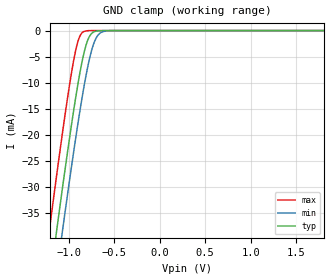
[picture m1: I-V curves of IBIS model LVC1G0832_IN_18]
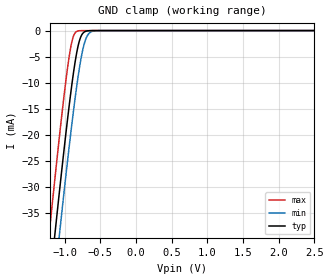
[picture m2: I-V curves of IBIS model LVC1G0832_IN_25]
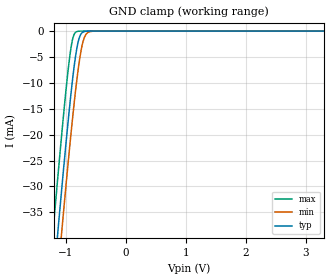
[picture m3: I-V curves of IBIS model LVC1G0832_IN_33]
| TEXAS INSTRUMENTS INCORPORATED
| Standard Linear and Logic Group
| IBIS Model of SN74LVC1G0832
| SINGLE 3-INPUT POSITIVE AND-OR GATE
| This file contains package information for the following:
|  SOT 5-pin (DBV) package as [Component] LVC1G0832_DBV
|  SOT 5-pin (DCK) package as [Component] LVC1G0832_DCK
|  NanoStar WCSP 5-pin (YEP) package as [Component] LVC1G0832_YEP
|  NanoFree WCSP 5-pin (YZP) package as [Component] LVC1G0832_YZP
| This device can be powered at the following Vccs:
|  1.8 volt Vcc
|  2.5 volt Vcc
|  3.3 volt Vcc
|  5 volt Vcc
| This file provides unique models under the [Model Selector] for each Vcc.
| For operation at a specific Vcc, select the appropriate model after each
| [Model Selector] keyword.
[IBIS Ver]   3.2
[Comment char]  |_char
[File Name]   sn74lvc1g0832.ibs
[File Rev]   1.2 | x_die
[Date]   August 4, 2005
[Source]   Data created from TI-SPICE simulations at TI-SLL.
[Notes]   The following is an IBIS list for the LVC1G0832.
   Please contact sllibis@ti.com with questions and
   comments concerning SLL IBIS models.
   - FILE REV HISTORY
   - 1.1 Release IBIS file on 10/04/04
   - 1.2 YEP and YZP packages added on 08/04/05
   - Due to the fact that the Device is 5.5-V Input tolarent,
   the pulldown model has some Non-Monotonic Warnings.
[Disclaimer] Property of Texas Instruments Incorporated.  Unauthorized
   reproduction and/or distribution is strictly prohibited.
   This product is protected under copyright law.
   Created  2004, (C) Copyright  2004, Texas Instruments
   Incorporated, All Rights Reserved
   UNLESS THERE IS A SIGNED, WRITTEN AGREEMENT TO THE
   CONTRARY, TEXAS INSTRUMENTS (TI) IS PROVIDING THE IBIS
   MODELS  AND WITHOUT ANY WARRANTY, EXPRESSED OR
   IMPLIED.  TI assumes no liability for:
   1) the accuracy of the IBIS models provided to your
   company;
   2) the proper functioning of these IBIS Models in your
   design or for any resulting applications; or
   3) infringement of patents, copyrights or intellectual
   property rights resulting from your use of these IBIS
   models.
   TI provides IBIS Models as a service to our customers.
   You and your company shall not distribute, sell or give
   these models to anyone else without prior written
   permission from TI.
   TI reserves the right to make changes to our products or
   to discontinue any semiconductor product or service
   without notice, and advises our customers to obtain the
   latest version of relevant information to verify, before
   placing orders, that the information being relied on is
   current.
   Please be aware that your receipt and use of the IBIS
   information provided shall serve as acceptance of these
   terms and conditions.  If you do not accept these terms,
   you should return or destroy the IBIS models and any
   other accompanying information immediately.
| Component LVC1G0832_DBV 5-pin SOT
[Component]   LVC1G0832_DBV
[Manufacturer]   Texas Instruments, Inc.
[Package]
|   typ   min   max
R_pkg   2.500e-02   1.900e-02   3.700e-02
L_pkg   1.524e-09   1.260e-09   1.751e-09
C_pkg   2.450e-13   1.980e-13   2.640e-13
[Pin]   signal_name   model_name   R_pin   L_pin   C_pin
1   A   LVC1G0832_IN   2.100e-02   1.405e-09   2.460e-13
2   B   LVC1G0832_IN   2.600e-02   1.493e-09   2.470e-13
3   GND   GND   3.700e-02   1.751e-09   2.630e-13
4   Y   LVC1G0832_OUT   1.900e-02   1.620e-09   2.640e-13
5   VCC   POWER   2.400e-02   1.260e-09   1.980e-13
| Component LVC1G0832_DCK 5-pin SOT
[Component]   LVC1G0832_DCK
[Manufacturer]   Texas Instruments, Inc.
[Package]
|   typ   min   max
R_pkg   2.500e-02   1.900e-02   3.700e-02
L_pkg   1.524e-09   1.260e-09   1.751e-09
C_pkg   2.450e-13   1.980e-13   2.640e-13
[Pin]   signal_name   model_name   R_pin   L_pin   C_pin
1   A   LVC1G0832_IN   2.100e-02   1.405e-09   2.460e-13
2   B   LVC1G0832_IN   2.600e-02   1.493e-09   2.470e-13
3   GND   GND   3.700e-02   1.751e-09   2.630e-13
4   Y   LVC1G0832_OUT   1.900e-02   1.620e-09   2.640e-13
5   VCC   POWER   2.400e-02   1.260e-09   1.980e-13
| Component LVC1G0832_YEP 5-pin NanoStar WCSP
[Component]   LVC1G0832_YEP
[Manufacturer]   Texas Instruments, Inc.
[Package]
|   typ   min   max
R_pkg   0.001   0.001   0.001
L_pkg   0.021nH   0.021nH   0.021nH
C_pkg   0.046pF   0.045pF   0.047pF
[Pin]   signal_name   model_name   R_pin   L_pin   C_pin
1   A   LVC1G0832_IN   0.001   0.021nH   0.046pF
2   B   LVC1G0832_IN   0.001   0.021nH   0.047pF
3   GND   GND   0.001   0.021nH   0.046pF
4   Y   LVC1G0832_OUT   0.001   0.021nH   0.045pF
5   VCC   POWER   0.001   0.021nH   0.045pF
| Component LVC1G0832_YZP 5-pin NanoStar WCSP
[Component]   LVC1G0832_YZP
[Manufacturer]   Texas Instruments, Inc.
[Package]
|   typ   min   max
R_pkg   0.001   0.001   0.001
L_pkg   0.021nH   0.021nH   0.021nH
C_pkg   0.046pF   0.045pF   0.047pF
[Pin]   signal_name   model_name   R_pin   L_pin   C_pin
1   A   LVC1G0832_IN   0.001   0.021nH   0.046pF
2   B   LVC1G0832_IN   0.001   0.021nH   0.047pF
3   GND   GND   0.001   0.021nH   0.046pF
4   Y   LVC1G0832_OUT   0.001   0.021nH   0.045pF
5   VCC   POWER   0.001   0.021nH   0.045pF
| Model LVC1G0832_IN
[Model Selector]   LVC1G0832_IN
LVC1G0832_IN_18   1.8 volt Vcc
LVC1G0832_IN_25   2.5 volt Vcc
LVC1G0832_IN_33   3.3 volt Vcc
LVC1G0832_IN_50   5 volt Vcc
| Model LVC1G0832_OUT
[Model Selector]   LVC1G0832_OUT
LVC1G0832_OUT_18   1.8 volt Vcc
LVC1G0832_OUT_25   2.5 volt Vcc
LVC1G0832_OUT_33   3.3 volt Vcc
LVC1G0832_OUT_50   5 volt Vcc
| Models and submodels in the file (8): LVC1G0832_IN_18 (Input), LVC1G0832_IN_25 (Input), LVC1G0832_IN_33 (Input), LVC1G0832_IN_50 (Input), LVC1G0832_OUT_18 (Output), LVC1G0832_OUT_25 (Output), LVC1G0832_OUT_33 (Output), LVC1G0832_OUT_50 (Output)
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[Model]   LVC1G0832_IN_18
Model_type  Input
Vinl=0.5775
Vinh=1.2675
| variable   typ   min   max
C_comp   3.51pF   2.98pF   4.34pF
[Temperature Range]   40   100   -40
| Ambient temperature   25   85   -40
[Voltage range]   1.8   1.65   1.95
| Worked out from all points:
|   GND clamp passes 1 mA (typ) near -0.77 V on its own axis
[GND Clamp]
| LVC1G0832_IN_18
|   Voltage   I(typ)   I(min)   I(max)
-5.5V     -655.2mA   -662.2mA   -646.6mA
-1.215V   -49.6mA    -57.88mA   -38.96mA
-1.135V   -39.07mA   -47.36mA   -28.42mA
-1.075V   -31.35mA   -39.6mA    -20.75mA
-1.055V   -28.82mA   -37.05mA   -18.27mA
-955mV    -16.68mA   -24.66mA   -6.874mA
-885mV    -9.098mA   -16.55mA   -1.486mA
-825mV    -3.922mA   -10.26mA   -137.1uA
-780mV    -1.472mA   -6.227mA   -17.15uA
-715mV    -205.4uA   -2.128mA   -808.5nA
-650mV    -22.01uA   -443.9uA   -37.93nA
1.8V      3.326pA    6.142pA    3.026pA
[Model]   LVC1G0832_IN_25
Model_type  Input
Vinl=0.7
Vinh=1.7
| variable   typ   min   max
C_comp   3.46pF   2.90pF   4.38pF
[Temperature Range]   40   100   -40
| Ambient temperature   25   85   -40
[Voltage range]   2.5   2.3   2.7
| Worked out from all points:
|   GND clamp passes 1 mA (typ) near -0.77 V on its own axis
[GND Clamp]
| LVC1G0832_IN_25
|   Voltage   I(typ)   I(min)   I(max)
-5.5V     -655.2mA   -662.2mA   -646.6mA
-1.215V   -49.6mA    -57.88mA   -38.96mA
-1.14V    -39.72mA   -48.01mA   -29.07mA
-1.12V    -37.12mA   -45.41mA   -26.48mA
-1.08V    -31.98mA   -40.25mA   -21.38mA
-1.06V    -29.44mA   -37.69mA   -18.89mA
-960mV    -17.26mA   -25.26mA   -7.377mA
-890mV    -9.597mA   -17.1mA    -1.734mA
-785mV    -1.671mA   -6.635mA   -21.67uA
-720mV    -242.5uA   -2.354mA   -1.023uA
-650mV    -22.01uA   -443.9uA   -37.93nA
2.5V      4.713pA    7.577pA    4.389pA
[Model]   LVC1G0832_IN_33
Model_type  Input
Vinl=0.8
Vinh=2.0
| variable   typ   min   max
C_comp   3.40pF   2.78pF   4.42pF
[Temperature Range]   40   100   -40
| Ambient temperature   25   85   -40
[Voltage range]   3.3   3   3.6
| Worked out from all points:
|   GND clamp passes 1 mA (typ) near -0.77 V on its own axis
[GND Clamp]
| LVC1G0832_IN_33
|   Voltage   I(typ)   I(min)   I(max)
-5.5V     -655.2mA   -662.2mA   -646.6mA
-1.225V   -50.93mA   -59.21mA   -40.3mA
-1.145V   -40.37mA   -48.66mA   -29.72mA
-1.12V    -37.12mA   -45.41mA   -26.48mA
-1.08V    -31.98mA   -40.25mA   -21.38mA
-1.06V    -29.44mA   -37.69mA   -18.89mA
-965mV    -17.84mA   -25.87mA   -7.89mA
-885mV    -9.098mA   -16.55mA   -1.486mA
-780mV    -1.472mA   -6.227mA   -17.15uA
-715mV    -205.4uA   -2.128mA   -808.5nA
-640mV    -15.53uA   -338.1uA   -23.69nA
3.3V      6.304pA    9.258pA    5.93pA
